VAR_GLOBAL CONSTANT
	
	cOversamples 	: UDINT 	:= 10;		            // number of oversamples
	
	cFFTLength		: UDINT		:= 2048;	            // length of FFT (power of 2)
	cWindowLength   : UDINT     := 2048;                // in this sample no zeropadding, but can be
	cBufferLength	: UDINT		:= cWindowLength/2;	    // buffer size; 50% overlap of windows
	cFFTResult 		: UDINT 	:= cFFTLength/2+1;  	// result of spectrum - cFFTLength/2+1
		
END_VAR
